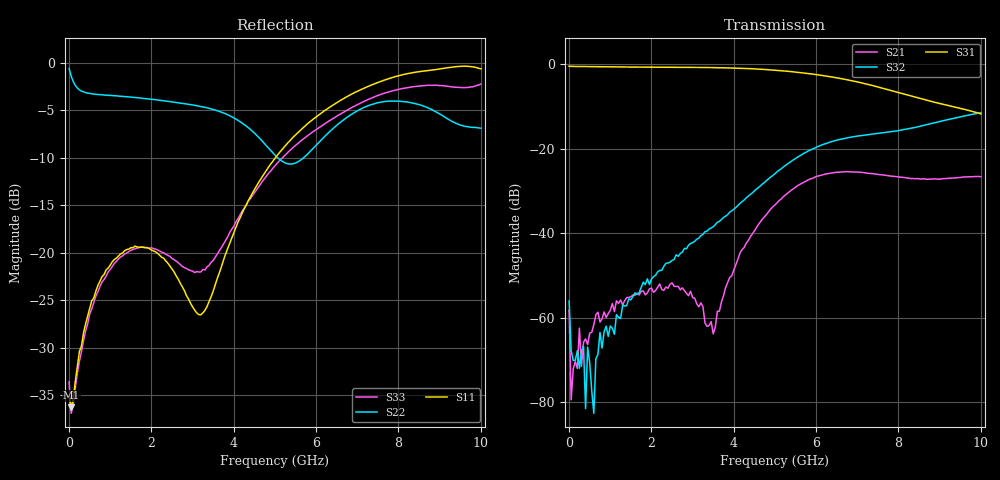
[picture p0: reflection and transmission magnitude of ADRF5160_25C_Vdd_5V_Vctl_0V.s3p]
! Device:  ADRF5160
! Description: Silicon SPDT Switch
! Frequency:  0.7 -  4 GHz
! Ports:
!	RFc	= Port 1
!	RF1	= Port 2
!  RF2  = Port 3
! Vdd:  5 Volt
! Control:  0 Volt
! Data:  Data was collected using a calibrated 4 port network analyzer and de-embedded using Agilent's AFR De-Embedding.
! Note:  Analog Devices supplies this data as a sample of measured data
!  for this product.  Your particular data for this product may vary.
!  Data was taken at 25 degrees C.
!  Analog Devices reserves the right to change this data at anytime.
!S3P File: Measurements: <S11,S12,S13>,
!<S21,S22,S23>,
!<S31,S32,S33>:
# Hz S  dB  R 50
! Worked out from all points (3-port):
!   201 points, 10 MHz to 10 GHz, reference 50 ohm
!   strongest paths, dB at 10 MHz, 2.507 GHz, 5.005 GHz, 7.503 GHz, 10 GHz:
!     S31: -0.5, -0.7, -1.4, -5.4, -11.8
!     S32: -56.0, -46.4, -25.9, -16.4, -11.5
!     S21: -58.3, -51.8, -33.3, -26.1, -26.6
!   lowest |S11| = -36.2 dB at 59.95 MHz (marker M1), VSWR 1.03, Z = 51.2 - j0.967 ohm
!   |S11| at or under -10 dB: start of sweep to 5.015 GHz
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1e7  -35.14 -17.0  -60.23 -51.3  -0.48 -0.4
     -58.31 -24.0  -0.63 -8.9  -56.07 168.7
     -0.45 -0.6  -56.04 -51.2  -33.58 -12.4
5.995e7  -36.24 -37.7  -61.48 -38.4  -0.51 -1.8
         -79.43 -117.6  -1.43 -45.8  -66.23 -55.3
         -0.50 -1.7  -67.83 -57.1  -36.88 -27.0
1.099e8  -35.40 -44.6  -78.92 -102.3  -0.50 -3.0
         -72.12 109.3  -1.99 -73.7  -63.41 47.4
         -0.51 -3.0  -70.14 54.8  -35.92 -50.6
2.5975e8  -30.38 -67.8  -65.96 41.4  -0.54 -6.9
          -62.49 91.7  -2.87 -122.2  -64.67 -63.4
          -0.53 -6.9  -71.96 28.8  -31.41 -77.3
3.097e8  -29.82 -75.5  -83.96 44.9  -0.53 -8.2
         -71.51 105.8  -3.00 -131.4  -77.17 89.6
         -0.54 -8.2  -67.86 -30.3  -30.39 -79.2
6.5935e8  -24.03 -91.6  -64.04 74.6  -0.56 -17.3
          -59.30 77.3  -3.33 -163.8  -65.93 -102.4
          -0.56 -17.3  -69.72 -78.5  -24.55 -101.0
3.5065e9  -24.02 85.8  -62.46 118.7  -0.79 -92.4
          -63.82 113.1  -4.93 119.6  -38.28 166.9
          -0.79 -92.4  -38.46 167.3  -20.80 -106.6
5.005e9  -10.05 10.4  -33.21 130.9  -1.40 -137.1
         -33.27 131.0  -9.73 106.2  -25.86 131.0
         -1.41 -137.0  -25.91 131.1  -10.86 -113.2
7.55245e9  -2.01 -50.5  -26.12 -10.7  -5.49 145.0
           -26.15 -10.6  -4.18 72.7  -16.32 15.6
           -5.50 145.1  -16.33 15.7  -3.37 156.0
1e10  -0.67 -79.3  -26.58 -76.7  -11.75 92.4
      -26.63 -76.6  -6.90 6.4  -11.46 -64.8
      -11.76 92.6  -11.46 -64.7  -2.26 83.4
